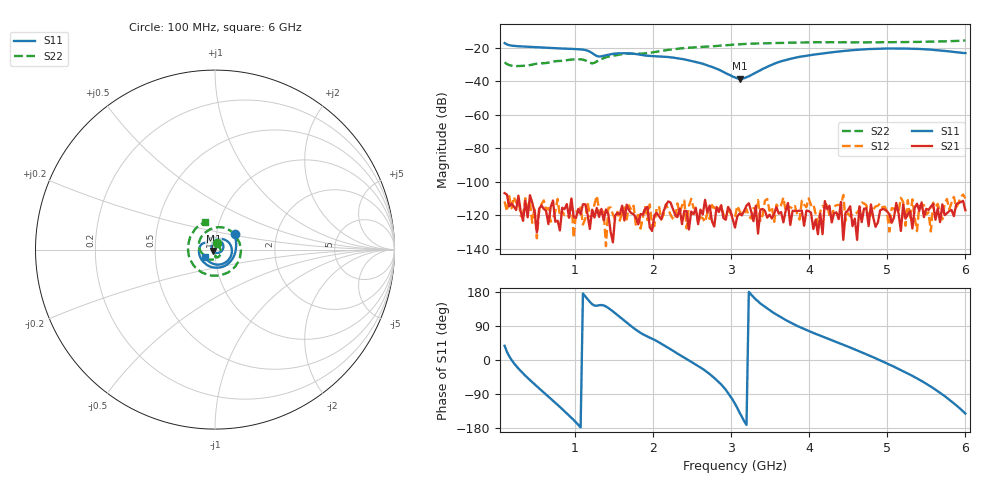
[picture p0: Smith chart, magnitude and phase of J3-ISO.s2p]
!Agilent Technologies,E8364B,MY43040379,A.07.50.67
!Agilent E8364B: A.07.50.67
!Date: Tuesday, March 24, 2026 10:44:23
!Correction: S11(Full 2 Port(1,2))
!S21(Full 2 Port(1,2))
!S12(Full 2 Port(1,2))
!S22(Full 2 Port(1,2))
!S2P File: Measurements: S11, S21, S12, S22:
# Hz S  dB  R 50
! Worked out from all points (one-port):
!   201 points, 100 MHz to 6 GHz, reference 50 ohm
!   lowest |S11| = -38.5 dB at 3.109 GHz (marker M1), VSWR 1.02, Z = 49.1 - j0.768 ohm
!   |S11| at or under -10 dB: start of sweep to end of sweep
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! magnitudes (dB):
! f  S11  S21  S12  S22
! 100 MHz  -17.2  -106.7  -111.7  -28.7
! 188.5 MHz  -18.7  -113.0  -115.7  -30.7
! 306.5 MHz  -19.2  -117.6  -120.4  -30.8
! 955.5 MHz  -20.7  -109.9  -110.0  -27.0
! 1.103 GHz  -21.1  -113.3  -125.4  -27.1
! 1.221 GHz  -23.1  -116.6  -120.3  -29.3
! 1.31 GHz  -25.2  -120.9  -116.7  -27.4
! 1.427 GHz  -24.1  -119.3  -115.5  -25.3
! 1.634 GHz  -23.3  -123.0  -115.2  -23.6
! 1.899 GHz  -24.6  -116.1  -114.2  -23.4
! 2.076 GHz  -25.1  -120.5  -114.5  -22.1
! 2.372 GHz  -26.7  -125.2  -114.1  -20.3
! 2.637 GHz  -29.5  -119.5  -121.6  -19.4
! 3.05 GHz  -37.7  -127.2  -121.1  -18.1
! 3.109 GHz  -38.5  -118.9  -117.3  -17.9
! 3.227 GHz  -37.0  -112.7  -120.4  -17.6
! 3.64 GHz  -28.1  -118.0  -113.9  -17.1
! 4.053 GHz  -24.1  -128.1  -113.0  -16.7
! 4.554 GHz  -21.4  -126.4  -119.0  -16.7
! 5.027 GHz  -20.4  -119.3  -129.6  -16.7
! 5.528 GHz  -21.0  -116.7  -118.1  -16.4
! 6 GHz  -23.2  -116.9  -109.8  -15.6
